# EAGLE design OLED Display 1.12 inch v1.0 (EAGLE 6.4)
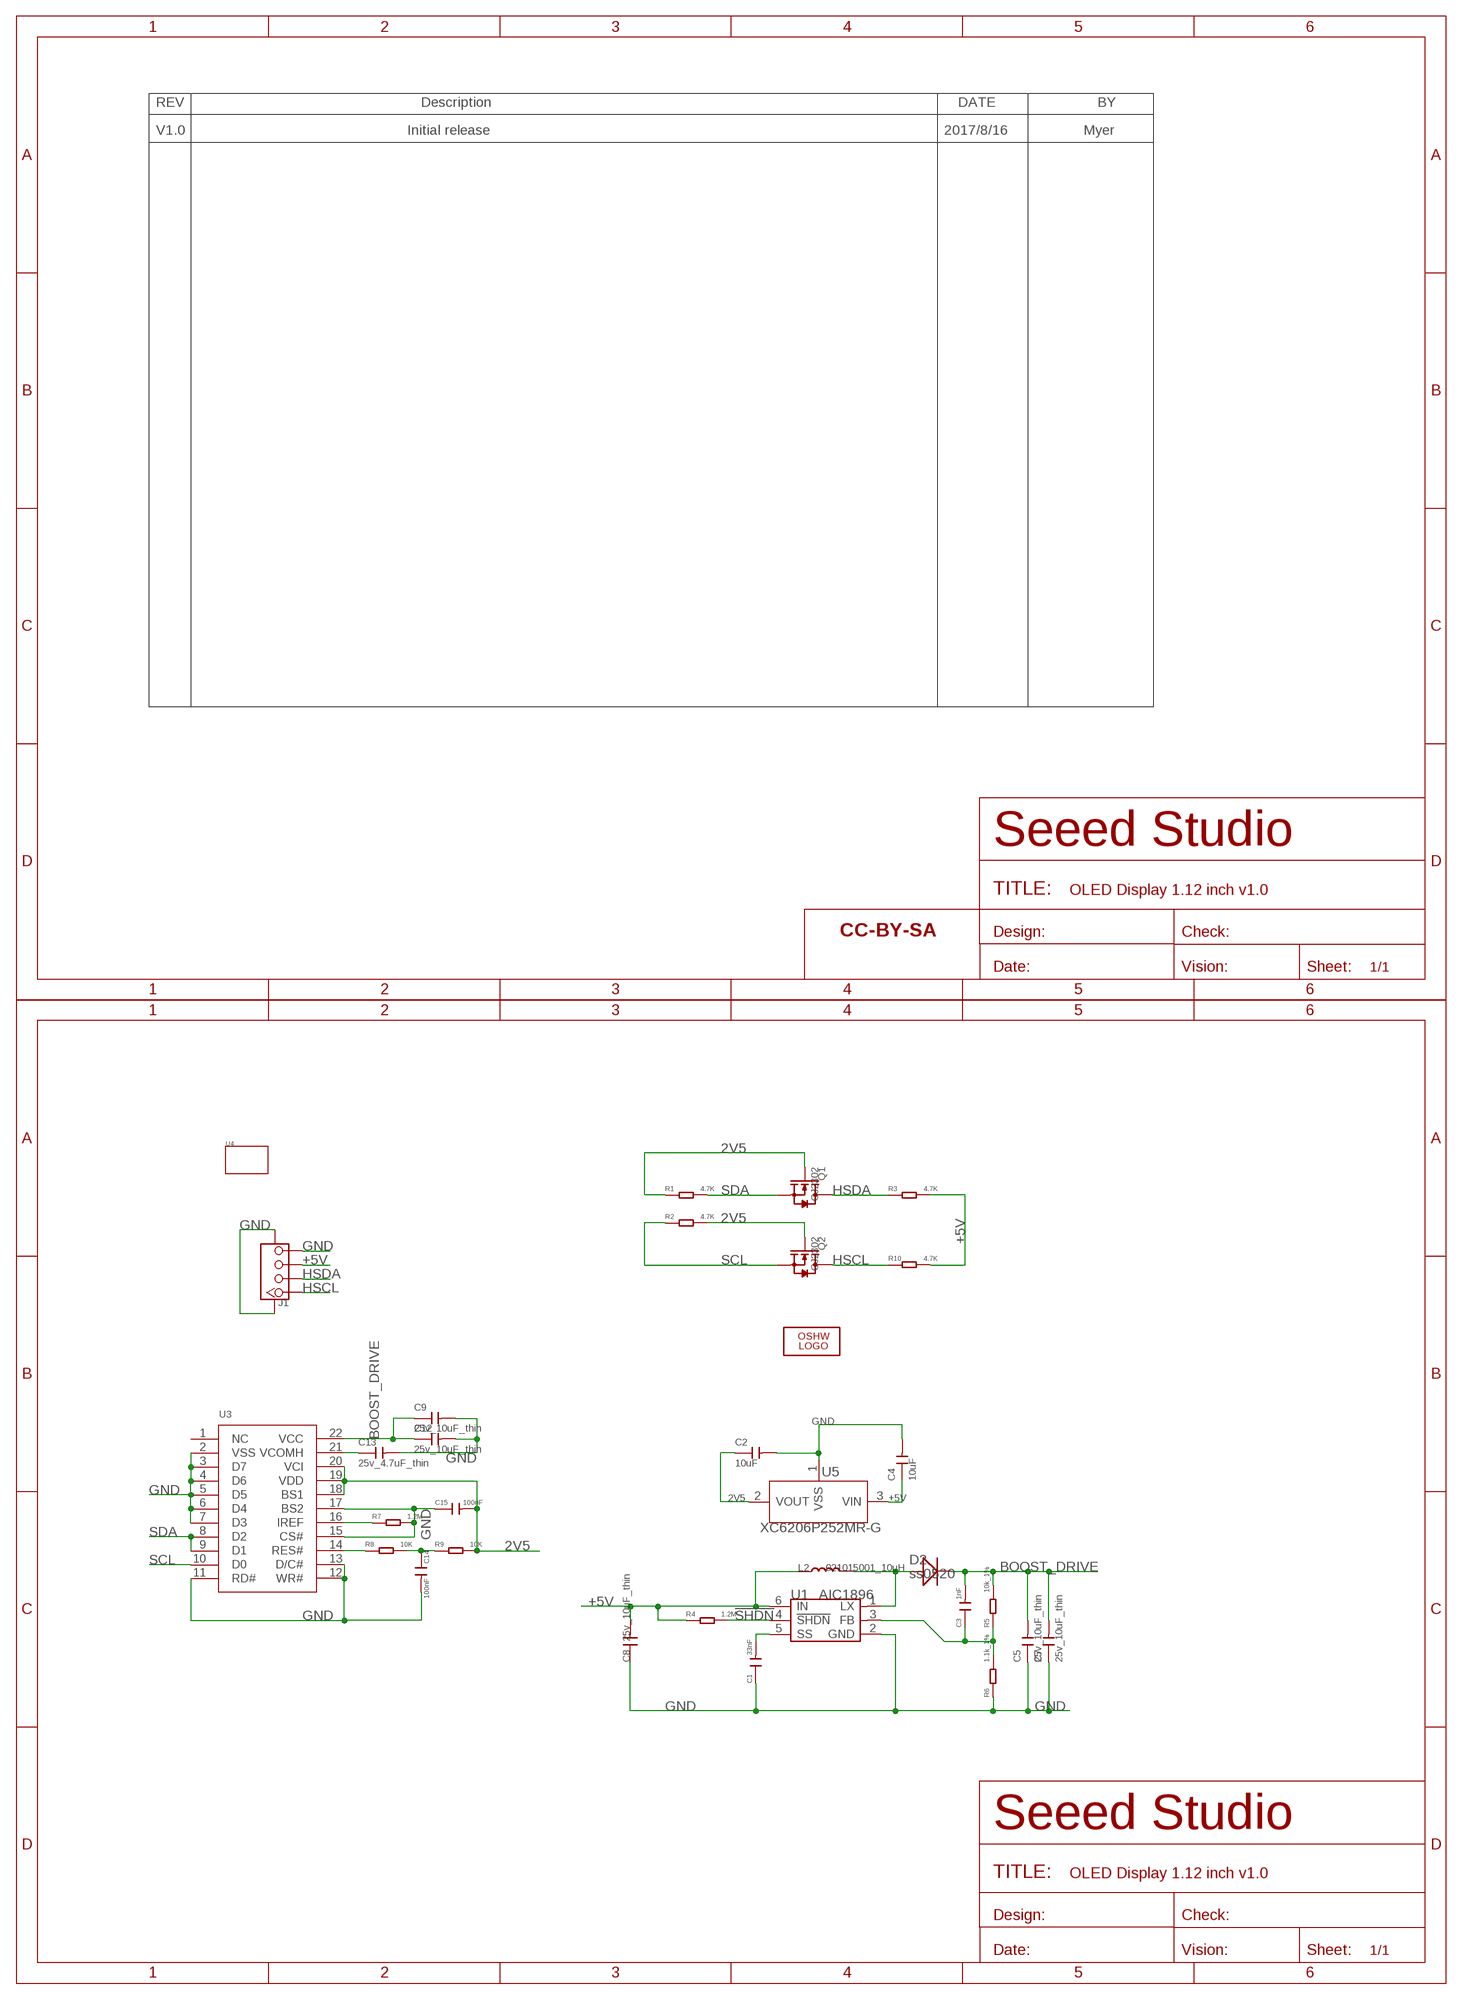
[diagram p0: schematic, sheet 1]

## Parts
C1  33nF  C-0402  [C0402]
C2  10uF  CAP-0603  [C0603]
C3  1nF  C-0402  [C0402]
C4  10uF  CAP-0603  [C0603]
C5  25v_10uF_thin  CAP-0805  [C0805]
C7  25v_10uF_thin  CAP-0805  [C0805]
C8  25v_10uF_thin  006-C0805  [0805]
C9  25v_10uF_thin  CAP-0805  [C0805]
C12  25v_10uF_thin  CAP-0805  [C0805]
C13  25v_4.7uF_thin  CAP-0805  [C0805]
C14  100nF  C-0402  [C0402]
C15  100nF  C-0402  [C0402]
D2  ss0520  010-DSOD123  [SOD123]
FR1  SEEEDSTUDIO-OPEN-SCH-FRAME  [SEEEDSTUDIO-PCB-FRAME]
J1  TWIG-4P-2.0-SMD-FEMALE-REINFORCE'90D'  [4P-SMD-2.0-90D]
L2  021015001_10uH  013-L0806  [0806]
LOGO2  LOGO-OSHW-FILLX0200-NT  [OSHW_FILLX200_NOTEXT]
Q1  CJ2302  MOSFET-N'SOT23'  [SOT23]
Q2  CJ2302  MOSFET-N'SOT23'  [SOT23]
R1  4.7K  R-0402  [R0402]
R2  4.7K  R-0402  [R0402]
R3  4.7K  R-0402  [R0402]
R4  1.2M  R-0402  [R0402]
R5  10k_1%  R-0402  [R0402]
R6  1.1k_1%  R-0402  [R0402]
R7  1.2M  R-0402  [R0402]
R8  10K  R-0402  [R0402]
R9  10K  R-0402  [R0402]
R10  4.7K  R-0402  [R0402]
U1  AIC1896  [SOT23-6]
U3  LCD22P-LY120-096096-PART  [LCD22P-SMD-0.7-30X27MM-PART]
U4  TWIG-2X2U  [2X2U-DIM-W/-DRILL]
U5  XC6206P252MR-G  XC6206MR  [SOT23]

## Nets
2V5: C2.1 C15.2 Q1.1(G) Q2.1(G) R1.1 R2.2 R9.2 U3.18(BS1) U3.19(VDD) U3.20(VCI) U5.2(VOUT)
!SHDN: R4.2 U1.4(!SHDN)
+5V: C4.1 C8.2 J1.3 L2.1 R3.2 R4.1 R10.2 U1.6(IN) U5.3(VIN)
BOOST_DRIVE: C3.2 C5.2 C7.2 C9.1 C12.1 D2.- R5.2 U3.22(VCC)
GND: C1.1 C2.2 C4.2 C5.1 C7.1 C8.1 C9.2 C12.2 C13.2 C14.2 C15.1 J1.4 J1.SS1 J1.SS2 R6.1 R7.2 U1.2(GND) U3.2(VSS) U3.3(D7) U3.4(D6) U3.5(D5) U3.6(D4) U3.7(D3) U3.11(RD#) U3.12(WR#) U3.13(D/C#) U3.15(CS#) U3.17(BS2) U5.1(VSS)
HSCL: J1.1 Q2.3(D) R10.1
HSDA: J1.2 Q1.3(D) R3.1
N$1: D2.+ L2.2 U1.1(LX)
N$2: C1.2 U1.5(SS)
N$4: C3.1 R5.1 R6.2 U1.3(FB)
N$9: C13.1 U3.21(VCOMH)
N$12: R7.1 U3.16(IREF)
N$19: R8.1 U3.14(RES#)
N$20: C14.1 R8.2 R9.1
SCL: Q2.2(S) R2.1 U3.10(D0)
SDA: Q1.2(S) R1.2 U3.8(D2) U3.9(D1)
Unconnected: U3.1(NC)

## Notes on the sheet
- V1.0 | Initial release | 2017/8/16 | Myer

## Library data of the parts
C1 C3 C14 C15 = Discrete-small:C*: Ceramic Capacitors
C2 C4 C5 C7 C9 C12 C13 = Discrete-new:CAP: Ceramic Capacitors
C8 = Discrete:006-C*: Ceramic Capacitors
D2 = Discrete:010-D*
FR1 = moudle-new:SEEEDSTUDIO-OPEN-SCH-FRAME
J1 = Connector:TWIG-4P-2.0-SMD-FEMALE-REINFORCE
L2 = Discrete:013-L*
LOGO2 = logo:LOGO-OSHW-FILL; PARTNO: DNP
Q1 Q2 = Discrete:MOSFET-N: IRLL014: http://www.vishay.com/docs/91319/sihll014.pdf
R1-R10 = Discrete-small:R*
U1 = ICs_v54:AIC1896
U3 = moudle-new:LCD22P-LY120-096096: 308010007
U4 = Module:TWIG
U5 = IC:XC6206: LOW ESR Cap.Compatible Positive Voltage Regulators

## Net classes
0 default: width 0.152 mm, drill 0.254 mm, clearance 0.152 mm

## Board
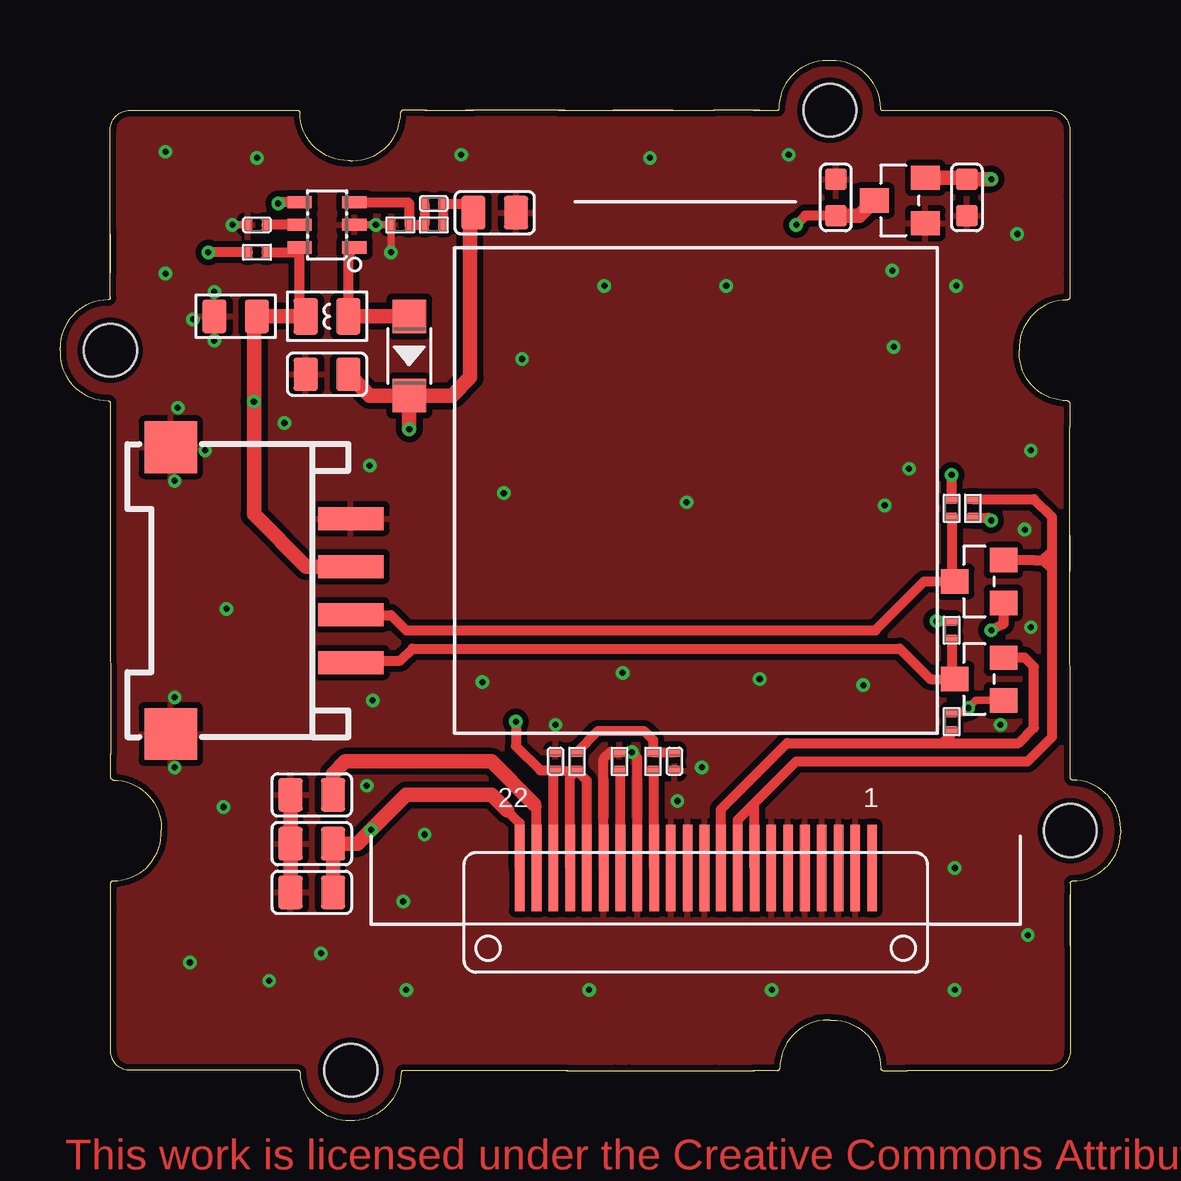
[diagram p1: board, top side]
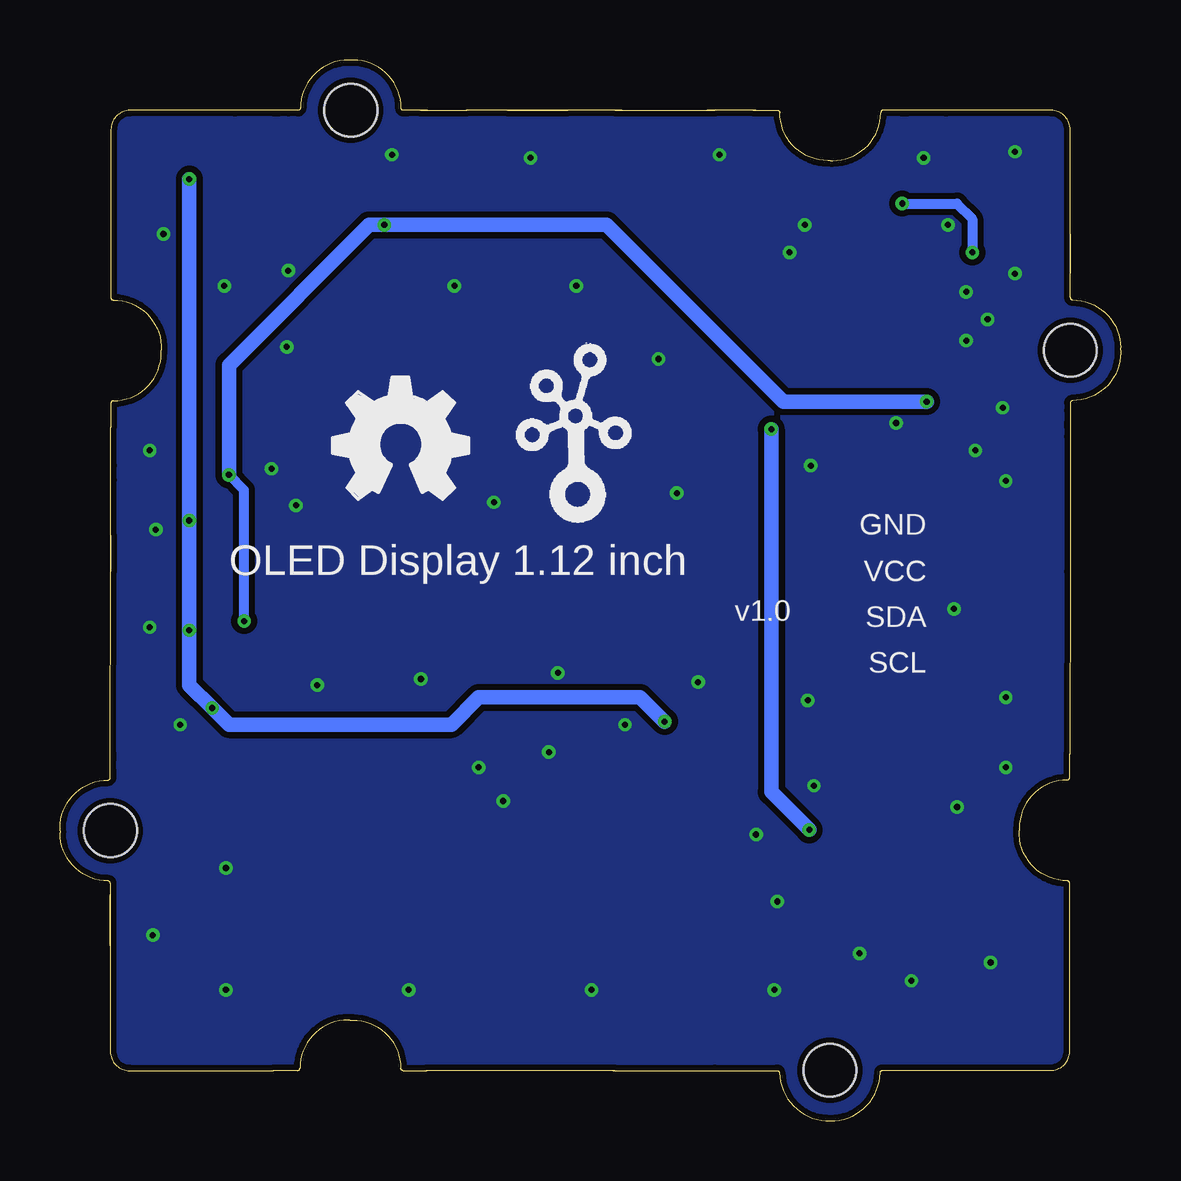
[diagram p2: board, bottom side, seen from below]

Size 44.21 x 44.2 mm. Coordinates in mm from the lower left corner, seen from the top.
Copper layers (1*16): Top 0.035mm / dielectric 1.5mm / Bottom 0.035mm
Design rules "SeeedStudio_2layer_DRU_no_angle_20140221 *": minimum track width 6mil, minimum drill 10mil, track to track 6mil, track to pad 6mil, pad to pad 6mil, via to via 6mil, smd to smd 0mil, copper to edge 10mil, drill to drill 10mil, minimum pad ring 10mil, minimum via ring 6mil, stop-mask expansion 2mil, vias tented up to drill 25mil, thermal gap 10mil
tRestrict: area 22.3,9 to 33.9,11.9

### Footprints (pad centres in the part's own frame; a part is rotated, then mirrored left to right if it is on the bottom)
C0402 = smd 0.508 x 0.385: 1 0,0.383; 2 0,-0.383
C0603 = smd 0.889 x 0.889: 1 0,0.762; 2 0,-0.762
C0805 = smd 1.397 x 1.016: 1 0,0.889; 2 0,-0.889
0805 = smd 1.016 x 1.397: 1 -0.889,0; 2 0.889,0
SOD123 = smd 1.397 x 1.397: + 1.651,0; - -1.651,0
4P-SMD-2.0-90D = smd 0.965 x 2.74: 1 -3,-0.1; 2 -1,-0.1; 3 1,-0.1; 4 3,-0.1 | smd 2.159 x 2.184: SS1 -5.974,7.4; SS2 5.974,7.4
0806 = smd 1.016 x 1.524: 1 -0.889,0; 2 0.889,0
SOT23 = smd 1.016 x 1.143: 1 -0.889,-1.016; 2 0.889,-1.016; 3 0,1.016
R0402 = smd 0.508 x 0.385: 1 0,0.383; 2 0,-0.383
SOT23-6 = smd 0.508 x 1.016: 1 -0.94,-1.143; 2 0,-1.143; 3 0.94,-1.143; 4 0.94,1.143; 5 0,1.143; 6 -0.94,1.143
LCD22P-SMD-0.7-30X27MM-PART = smd 0.4 x 3.6: 1 7.35,-12.7; 2 6.65,-12.7; 3 5.95,-12.7; 4 5.25,-12.7; 5 4.55,-12.7; 6 3.85,-12.7; 7 3.15,-12.7; 8 2.45,-12.7; 9 1.75,-12.7; 10 1.05,-12.7; 11 0.365,-12.7; 12 -0.335,-12.7; 13 -1.035,-12.7; 14 -1.735,-12.7; 15 -2.435,-12.7; 16 -3.135,-12.7; 17 -3.835,-12.7; 18 -4.535,-12.7; 19 -5.235,-12.7; 20 -5.935,-12.7; 21 -6.635,-12.7; 22 -7.335,-12.7
2X2U-DIM-W/-DRILL = hole 2.2: 10.033,20.01; -19.955,10.015; -9.933,-19.99; 20.055,-9.995
SOT23' = smd 1.016 x 1.2: 1 -0.95,-1.06; 2 0.95,-1.06; 3 0,1.06

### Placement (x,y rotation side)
C1  8.21,37.33 90 top
C2  37.8,38.47 0 top
C3  15.58,38.22 90 top
C4  32.34,38.47 180 top
C5  18.12,37.84 270 top
C7  11.13,31.11 90 top
C8  7.32,33.52 0 top
C9  10.5,9.52 270 top
C12  10.5,11.55 270 top
C13  10.5,13.58 270 top
C14  25.61,14.98 0 top
C15  20.66,14.98 0 top
D2  14.56,31.87 90 top
FR1  not placed on the board
J1  12.02,22.09 90 top
L2  11.13,33.52 0 top
LOGO2  32.85,25.9 0 bottom
Q1  38.31,22.47 90 top
Q2  38.31,18.41 90 top
R1  38.06,25.52 180 top
R2  37.17,16.63 180 top
R3  37.17,25.52 180 top
R4  8.21,36.19 270 top
R5  15.58,37.33 90 top
R6  14.18,37.33 90 top
R7  23.32,14.98 180 top
R8  24.72,14.98 180 top
R9  21.55,14.98 0 top
R10  37.17,20.44 180 top
U1  11.13,37.33 90 top
U3  26.5,23.23 0 top
U4  22.05,22.09 0 top
U5  XC6206P252MR-G  [SOT23']  35.01,38.35 90 top
U$1  [TWIGLOGO]  22.69,25.9 0 bottom

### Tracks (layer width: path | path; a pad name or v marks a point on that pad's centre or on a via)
2V5  (via drill 0.25 pad 0.51)
  Top 0.305: Q2.1 38.18,17.52 v37.87,17.2 37.68,17.01 R2.2
  Top 0.406: U3.20 20.57,14.5 C15.2 | U3.18 21.96,14.18 R9.2 | U3.19 21.27,14.31 R9.2 | C15.2 R9.2 | v19.01,16.63 19.01,15.61 20.02,14.6 C15.2 | R1.1 38.69,25.14 v38.82,25.01 | Q1.1 39.33,20.69 v38.82,20.44
  Top 0.61: U5.2 37.74,39.3 C2.1 v38.82,39.23
  Bottom 0.61: v38.82,39.23 v38.82,25.01 v38.82,20.44 38.82,18.16 v37.87,17.2 37.17,16.5 27.89,16.5 26.75,17.64 20.02,17.64 v19.01,16.63
!SHDN  (via drill 0.25 pad 0.51)
  Top 0.406: R4.2 v6.18,36.19 | U1.4 9.15,38.27 v9.1,38.22
  Bottom 0.406: v9.1,38.22 6.81,38.22 6.18,37.58 v6.18,36.19
+5V  (via drill 0.25 pad 0.51)
  Top 0.406: L2.1 9.99,33.77 U1.6 9.79,36.19 R4.1 | v30.69,37.33 31.07,37.71 C4.1 | R3.2 v37.17,26.92 | R10.2 v36.53,20.82
  Top 0.61: L2.1 C8.2 8.08,33.39 v8.08,29.96 8.08,25.26 10.26,23.09 J1.3 | C4.1 33.31,37.71 U5.3
  Bottom 0.406: v36.53,20.82 36.53,26.28 v37.17,26.92
  Bottom 0.61: v8.08,29.96 14.05,29.96 21.42,37.33 v30.69,37.33 31.33,37.33 37.17,31.49 v37.17,26.92
BOOST_DRIVE  (via drill 0.25 pad 0.51)
  Top 0.406: R5.2 C3.2 16.85,38.22 C5.2 | U3.22 19.16,12.41 18.31,13.26
  Top 0.61: C9.1 C12.1 12.4,11.55 12.91,12.06 v12.97,12.12 14.43,13.58 17.99,13.58 18.31,13.26 18.63,12.95 | D2.- 12.91,30.22 C7.2 | D2.- 16.34,30.22 17.1,30.98 17.1,37.71 C5.2 | D2.- v14.56,28.82
  Bottom 0.61: v14.56,28.82 14.56,13.71 v12.97,12.12
GND  (via drill 0.25 pad 0.51)
  Top 0.305: C1.1 v7.2,37.33 | v13.8,36.19 R6.1 v13.16,37.33 U1.2
  Top 0.406: U3.15 24.06,15.13 v23.83,15.36 | U3.17 22.66,15.08 22.94,15.36 R7.2
  Top 0.61: C9.2 C12.2 C13.2
  other vias: 5.54,33.39 6.43,32.5 6.43,34.54 13.04,17.52 8.21,40.12 4.91,29.71 6.05,27.93 4.78,26.66 4.78,17.64 39.2,16.5 4.78,14.72 5.42,6.6 10.88,6.98 14.31,9.14 20.66,16.5 8.72,5.83 25.74,13.33 26.75,14.72 30.37,40.25 34.69,35.42 37.36,34.79 39.9,36.95 23.45,18.66 17.61,18.28 33.48,18.15 40.47,27.93 40.34,7.74 37.3,10.53 37.3,5.45 29.68,5.45 22.05,5.45 14.43,5.45 29.17,18.41 6.81,13.07 6.94,21.33 40.47,20.57 4.4,35.3 4.4,40.38 16.72,40.25 24.59,40.12 12.91,27.3 34.37,25.65 27.77,34.79 22.69,34.79 18.5,26.15 26.12,25.77 12.78,13.96 19.26,31.74 35.39,27.17 34.75,32.25 15.2,11.93 40.22,24.63 9.36,29.07
  pour Top (isolate 0.254, rank 2): -0.17,-0.14 44.28,0.25 44.28,44.7 -0.17,44.31
  pour Bottom (isolate 0.254, rank 6): -0.17,-0.14 44.28,-0.14 44.28,44.31 -0.17,44.31
HSCL
  Top 0.406: 12.17,19.04 J1.1 12.2,19.17 14.18,19.17 14.69,19.68 35.01,19.68 36.28,18.41 Q2.3 37.17,18.53 R10.1
HSDA
  Top 0.406: J1.2 12.14,21.07 13.8,21.07 14.43,20.44 33.99,20.44 36.02,22.47 Q1.3 | 37.17,22.34 Q1.3 | R3.1 37.17,22.6 Q1.3
N$1
  Top 0.406: L2.2 12.02,36.14 U1.1
  Top 0.61: D2.+ L2.2
N$2
  Top 0.406: U1.5 C1.2
N$4
  Top 0.406: U1.3 14.51,38.27 14.56,38.22 R6.2 R5.1 C3.1
N$9
  Top 0.406: U3.21 19.86,13.1 19.77,13.2
  Top 0.61: 19.77,13.2 17.99,14.98 11.89,14.98 11.39,14.47 C13.1
N$12
  Top 0.406: U3.16 23.36,14.55 R7.1
N$19
  Top 0.406: U3.14 24.77,14.55 R8.1
N$20
  Top 0.406: R9.1 22.44,16.25 24.34,16.25 24.72,15.87 R8.2 C14.1
SCL
  Top 0.406: U3.10 27.55,12.98 30.31,15.74 36.79,15.74 | 36.79,15.74 39.96,15.74 40.6,16.38 40.6,18.91 40.22,19.3 Q2.2 | R2.1 37.17,16.12 36.79,15.74
SDA
  Top 0.406: U3.8 28.95,13.24 | 28.95,13.24 30.69,14.98 40.34,14.98 41.36,15.99 41.36,22.98 | 41.36,23.36 40.98,23.36 | Q1.2 40.6,23.36 40.98,23.36 | U3.9 28.25,12.54 28.95,13.24 | 41.36,22.98 41.36,23.36 | 41.36,23.36 41.36,23.74 | 41.36,23.74 41.36,25.14 40.59,25.9 R1.2 | 40.98,23.36 41.36,23.74 | 40.98,23.36 41.36,22.98

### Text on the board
bPlace: GND | VCC | OLED Display 1.12 inch | SDA | v1.0 | SCL

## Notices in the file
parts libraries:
moudle-new: This work is licensed under the Creative Commons Attribution 4.0 International License.
To view a copy of this license,visit:
http://creativecommons.org/licenses/by-sa/4.0
moudle-new: CC-BY-SA
